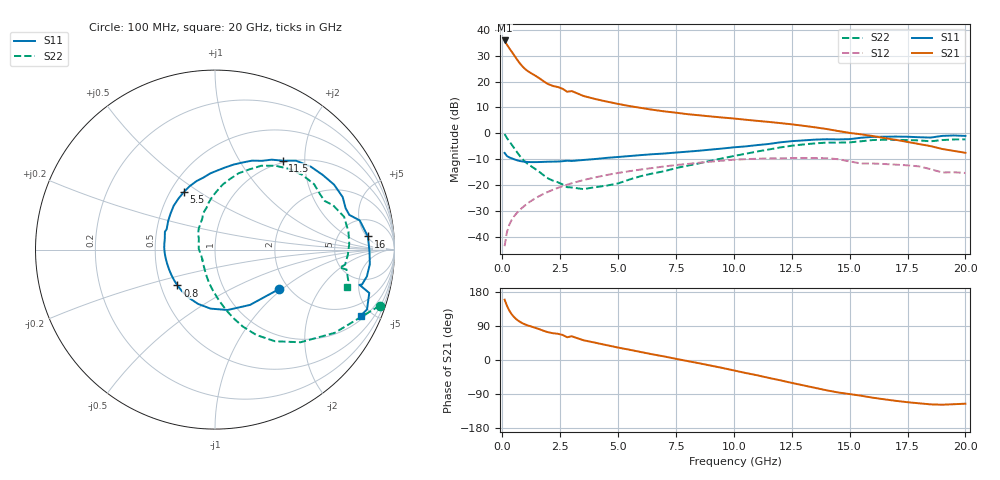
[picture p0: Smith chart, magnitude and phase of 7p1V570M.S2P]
! Infineon Technologies  Discrete & RF Semiconductors
! bfp620
! VCE =  1.5 V,  IC =  70 mA
! Common Emitter S-Parameters:  Sep 2002
# GHz  S  MA  R  50
!  f  S11  S21  S12  S22
! GHz  MAG  ANG  MAG  ANG  MAG  ANG  MAG  ANG
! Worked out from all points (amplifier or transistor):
!   59 points, 100 MHz to 20 GHz, reference 50 ohm
!   highest |S21| = 35.9 dB at 100 MHz (marker M1)
!   |S21| within 3 dB of that: start of sweep to 301.2 MHz
!   unconditionally stable (mu >= 1): 2.104 GHz to 2.233 GHz; 3.086 GHz to 9.912 GHz; 17.15 GHz to end of sweep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
!   at 1 GHz: K = 0.89, MSG = 26.2 dB, |S12| = -27.7 dB
!   at 5.5 GHz: K = 1.04, MAG = 11.4 dB, |S12| = -14.6 dB
!   at 20 GHz: K = 1.31, MAG = 0.6 dB, |S12| = -15.3 dB
!   S11 on the Smith chart (normalised r, x): 100 MHz: 1.78, -0.95; 800 MHz: 0.61, -0.27; 5.5 GHz: 0.58, +0.43; 11.5 GHz: 0.97, +1.57; 16 GHz: 10, +5; 20 GHz: 1.20, -4.31
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0.1  0.4187 -31.8  62.39 159.2  0.0066 80.5  0.9697 -18.8
0.2  0.3647 -57.7  51.65 143.3  0.0123 72.8  0.8124 -34.8
0.3  0.3437 -78.2  44.24 130.7  0.017 69.8  0.7025 -47.3
0.4  0.3298 -94.3  38.18 121.1  0.021 68.1  0.6104 -56.8
0.5  0.3169 -107.4  32.87 113.8  0.0246 67.0  0.5281 -64.2
0.6  0.3054 -118.6  28.27 108.0  0.0279 66.3  0.4559 -70.1
0.7  0.2962 -128.2  24.43 103.2  0.0312 65.8  0.395 -75.0
0.8  0.2894 -136.3  21.38 99.4  0.0345 65.4  0.346 -79.2
0.9  0.2847 -143.0  19.04 96.2  0.0378 65.1  0.308 -82.8
1.1  0.2796 -153.2  15.97 91.3  0.0445 64.5  0.2565 -88.7
1.9  0.2824 179.7  9.398 74.7  0.0715 59.7  0.1422 -111.3
2.8  0.2963 160.4  6.367 60.0  0.1018 52.1  0.0912 -141.1
3  0.2923 157.2  6.556 62.6  0.1085 50.3  0.09 -140.0
3.5  0.3057 148.6  5.286 52.2  0.1249 45.5  0.0836 -160.4
5.5  0.3642 118.8  3.36 27.0  0.186 25.6  0.1285 137.2
7  0.4073 98.8  2.66 9.3  0.2293 10.7  0.1853 112.6
10.5  0.5591 62.2  1.835 -34.2  0.3172 -29.4  0.4021 78.0
11.5  0.6229 52.7  1.664 -47.1  0.3289 -41.8  0.4862 66.8
13.5  0.7558 28.6  1.309 -73.4  0.3323 -65.8  0.6397 40.7
16  0.855 4.9  0.887 -99.5  0.2614 -89.6  0.7424 14.2
17  0.8664 -5.4  0.748 -107.8  0.2485 -97.5  0.7485 2.4
20  0.8915 -24.4  0.421 -115.3  0.1719 -107.3  0.7649 -15.9
